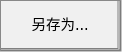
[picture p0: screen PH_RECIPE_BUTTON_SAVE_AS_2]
VISUALIZATION PH_RECIPE_BUTTON_SAVE_AS_2  // 122x52
VAR_IN_OUT
	RECIPE_CTRL_V2 : ST_RecipeCtrl_2;
END_VAR
    Button (0,0 120x50), "另存为...", input disabled if: (RECIPE_CTRL_V2.sStatus.bBusy) <> 0, text list: 'TextList_Recipe', text index: 113
        p55702900: SEL(RECIPE_CTRL_V2.sCmd.bRecipeSaveAs, 16#000000, 16#00FF00)
        tap RECIPE_CTRL_V2.sCmd.bRecipeSaveAs
END_VISUALIZATION
